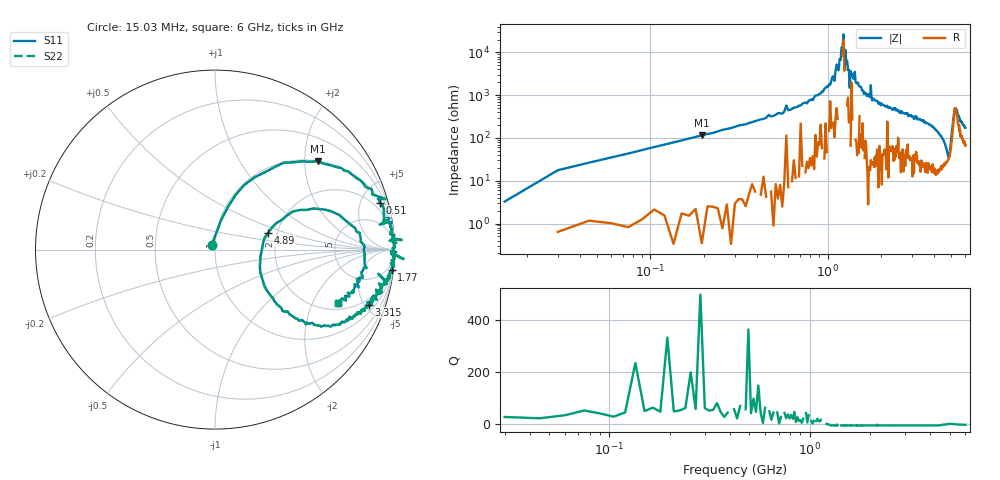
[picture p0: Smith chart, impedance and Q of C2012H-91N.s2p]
!	Network	Analyzer	HP8753E.07.74:	Oct	30	2002	Serial	No.	JP38451487
!	Hewlett-Packard
!	28	Aug	2009	10:30:47
!	Frequency	S11	S21	S12	S22
#	HZ	S	RI	R	50
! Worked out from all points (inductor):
!   400 points, 15.03 MHz to 6 GHz, reference 50 ohm
!   read as one part in series: L = 92.5 nH near 45.03 MHz
!   highest Q = 62.5 at 195 MHz (marker M1), where L = 94.8 nH
!   self-resonance near 1.215 GHz
!   S11 on the Smith chart (normalised r, x): 15.03 MHz: 0.96, +0.05; 510 MHz: 1.17, +6.99; 1.77 GHz: 2, -18; 3.315 GHz: 1.49, -5.35; 4.89 GHz: 1.79, +0.37; 6 GHz: 2.36, -3.19
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1.502992e7  -0.0177 0.0273  1.02 -0.0273  1.02 -0.0273  -0.0177 0.0273
3.002985e7  0.0359 0.169  0.964 -0.169  0.964 -0.169  0.0359 0.169
4.502978e7  0.0747 0.242  0.925 -0.242  0.925 -0.242  0.0747 0.242
1.95029e8  0.574 0.493  0.426 -0.493  0.426 -0.493  0.574 0.493
5.100274e8  0.919 0.261  0.0809 -0.261  0.0809 -0.261  0.919 0.261
1.020025e9  0.992 0.0547  0.00751 -0.0547  0.00751 -0.0547  0.992 0.0547
1.155024e9  0.999 0.0262  0.000672 -0.0262  0.000672 -0.0262  0.999 0.0262
1.230024e9  0.997 -0.00256  0.00281 0.00256  0.00281 0.00256  0.997 -0.00256
1.245024e9  0.98 -0.0113  0.0196 0.0113  0.0196 0.0113  0.98 -0.0113
1.260024e9  0.997 -0.00809  0.00305 0.00809  0.00305 0.00809  0.997 -0.00809
1.335023e9  1.05 -0.0524  -0.048 0.0524  -0.048 0.0524  1.05 -0.0524
1.350023e9  0.999 -0.0271  0.00122 0.0271  0.00122 0.0271  0.999 -0.0271
1.425023e9  1 -0.0284  -0.00164 0.0284  -0.00164 0.0284  1 -0.0284
1.770021e9  0.984 -0.112  0.0159 0.112  0.0159 0.112  0.984 -0.112
2.01002e9  0.967 -0.151  0.033 0.151  0.033 0.151  0.967 -0.151
3.015015e9  0.902 -0.278  0.0978 0.278  0.0978 0.278  0.902 -0.278
3.315013e9  0.857 -0.307  0.143 0.307  0.143 0.307  0.857 -0.307
4.00501e9  0.72 -0.406  0.28 0.406  0.28 0.406  0.72 -0.406
4.890006e9  0.295 0.0925  0.705 -0.0925  0.705 -0.0925  0.295 0.0925
5.010005e9  0.547 0.229  0.453 -0.229  0.453 -0.229  0.547 0.229
5.235004e9  0.834 0.0169  0.166 -0.0169  0.166 -0.0169  0.834 0.0169
6e9  0.687 -0.297  0.313 0.297  0.313 0.297  0.687 -0.297
